|Texas Instruments Incorporated
|16-Channel LED Driver w/EEprom DOT Correction & Grayscale PWM Control
| Marketing part#   Digital Voltage Range   Package-type   #pins
| TLC5940NT   3.0 to 5.5V   PDIP   28
| TLC5940NTG4   3.0 to 5.5V   PDIP   28
| TLC5940PWP   3.0 to 5.5V   HTSSOP   28
| TLC5940PWPG4   3.0 to 5.5V   HTSSOP   28
| TLC5940PWPR   3.0 to 5.5V   HTSSOP   28
| TLC5940PWPRG4   3.0 to 5.5V   HTSSOP   28
| TLC5940RHBR   3.0 to 5.5V   QFN   32
| TLC5940RHBRG4   3.0 to 5.5V   QFN   32
[IBIS Ver]   3.2
[File name]   tlc5940.ibs
|SIMDE Ver   V2.0 - 201002 - RHL4 - Build 372
[File Rev]   1.0
[Date]   9/8/2010
[Source]
| Texas Instruments Incorporated.
| Analog-eLab Design Center, HPA
| 12500 TI Blvd
| Dallas, TX -75243
| e-mail: elab_ibis@list.ti.com
| -Model generated from simulations in TISPICE
[Notes]   Revision History:
| Rev 1.0: 9/8/2010
| - Initial version of the model
| - Model generated from simulations in TISPICE
| - Model matched to SPICE simulation
| - C_comp although listed in numerical order of value are
|   obtained from varying PVT conditions. For PVT conditions for
|   each specific value refer the buffer description under
|   respective [Model]. IBIS model user is responsible for using
|   appropriate C_comp to simulate for Signal Integrity.
[Disclaimer]
| This model is designed as an aid for customers of Texas Instruments.
| TI and its licensors and suppliers make no warranties, either expressed
| or implied, with respect to this  model, including the warranties of
| merchantability or fitness for a particular purpose. The model is
| provided solely on an "as is" basis. The entire risk as to its quality
| and performance is with the customer.
[Copyright]
 (C) Copyright 2010 Texas Instruments Incorporated.All rights reserved.
|   TLC5940PWP
[Component]   TLC5940PWP
[Manufacturer]   TI
[Package]   |28 HTSSOP -  PWP package
|   typ   min   max
R_pkg   0.08193   0.05437   0.11416
L_pkg   2.86912nH   2.09991nH   4.18774nH
C_pkg   0.49015pF   0.4277pF   0.62179pF
[Pin]  signal_name   model_name   R_pin   L_pin   C_pin
1   GND   GND   0.04408   3.68717nH  0.70954pF
2   BLANK   INPUT   0.11352   3.84749nH  0.5889pF
3   XLAT   INPUT   0.09801   3.15255nH  0.48789pF
4   SCLK   INPUT   0.08218   2.76394nH  0.47901pF
5   SIN   INPUT   0.06987   2.46426nH  0.45688pF
6   VPRG   TERM   0.06162   2.27164nH  0.43906pF
7   OUT0   TERM   0.05581   2.13231nH  0.42984pF
8   OUT1   TERM   0.05437   2.09991nH  0.42781pF
9   OUT2   TERM   0.05967   2.23421nH  0.43955pF
10   OUT3   TERM   0.06917   2.45494nH  0.45622pF
11   OUT4   TERM   0.08271   2.78637nH  0.47877pF
12   OUT5   TERM   0.09792   3.16124nH  0.48694pF
13   OUT6   TERM   0.11416   3.87798nH  0.58872pF
14   OUT7   TERM   0.11147   4.18774nH  0.62179pF
15   OUT8   TERM   0.11145   4.18614nH  0.62137pF
16   OUT9   TERM   0.11411   3.87312nH  0.58858pF
17   OUT10   TERM   0.09792   3.16127nH  0.48694pF
18   OUT11   TERM   0.08271   2.78627nH  0.4788pF
19   OUT12   TERM   0.06917   2.45496nH  0.45621pF
20   OUT13   TERM   0.05967   2.23422nH  0.43953pF
21   OUT14   TERM   0.05437   2.10017nH  0.4277pF
22   OUT15   TERM   0.05581   2.13233nH  0.42914pF
23   XERR   XERR   0.06071   2.24986nH  0.43618pF
24   SOUT   OUTPUT   0.06752   2.4073nH   0.45212pF
25   GSCLK   INPUT   0.07954   2.69933nH  0.47442pF
26   DCPRG   INPUT   0.09534   3.08672nH  0.48741pF
27   IREF   TERM   0.11132   3.79072nH  0.58402pF
28   VCC   POWER   0.1141   4.23499nH  0.6181pF
|   TLC5940RHB
[Component]   TLC5940RHB
[Manufacturer]   TI
[Package]   |32 QFN -  RHB package
|   typ   min   max
R_pkg   0.08145   0.00024   0.10927
L_pkg   1.45259nH   0.05657nH   1.97475nH
C_pkg   0.13023pF   0.04173pF   0.1566pF
[Pin]  signal_name   model_name   R_pin   L_pin   C_pin
1   SCLK   INPUT   0.10683   1.92034nH  0.15309pF
2   SIN   INPUT   0.10002   1.78371nH  0.15428pF
3   VPRG   TERM   0.09526   1.68977nH  0.14836pF
4   OUT0   TERM   0.09177   1.62167nH  0.14501pF
5   OUT1   TERM   0.09085   1.60457nH  0.14424pF
6   OUT2   TERM   0.0945   1.67768nH  0.14872pF
7   OUT3   TERM   0.10082   1.8039nH   0.1566pF
8   OUT4   TERM   0.10927   1.97475nH  0.15632pF
9   OUT5   TERM   0.10077   1.80744nH  0.14432pF
10   OUT6   TERM   0.0827   1.44881nH  0.13242pF
11   OUT7   TERM   0.07284   1.25667nH  0.11872pF
12   NC   NC   0.00024   0.05657nH  0.04173pF
13   NC   NC   0.00024   0.05657nH  0.04173pF
14   OUT8   TERM   0.07284   1.25667nH  0.11872pF
15   OUT9   TERM   0.0827   1.4489nH   0.13243pF
16   OUT10   TERM   0.10077   1.80745nH  0.14432pF
17   OUT11   TERM   0.10927   1.97474nH  0.15632pF
18   OUT12   TERM   0.10082   1.80391nH  0.1566pF
19   OUT13   TERM   0.0945   1.67767nH  0.14871pF
20   OUT14   TERM   0.09085   1.60457nH  0.14418pF
21   OUT15   TERM   0.09177   1.62167nH  0.14416pF
22   XERR   XERR   0.09456   1.67617nH  0.14589pF
23   SOUT   OUTPUT   0.09812   1.7463nH   0.15114pF
24   GSCLK   INPUT   0.10453   1.87495nH  0.15048pF
25   DCPRG   INPUT   0.09727   1.72964nH  0.14393pF
26   IREF   TERM   0.07733   1.33561nH  0.12703pF
27   VCC   POWER   0.07581   1.30567nH  0.11952pF
28   NC   NC   0.00024   0.05657nH  0.04173pF
29   NC   NC   0.00024   0.05657nH  0.04173pF
30   GND   GND   0.026   0.97478nH  0.17132pF
31   BLANK   INPUT   0.08126   1.4124nH   0.13077pF
32   XLAT   INPUT   0.10039   1.79135nH  0.1433pF
|   TLC5940NT
[Component]   TLC5940NT
[Manufacturer]   TI
[Package]   |28 PDIP - NT package
|   typ   min   max
R_pkg   0.09933   0.05587   0.11678
L_pkg   9.80714nH   4.19963nH   14.18524nH
C_pkg   1.93393pF   0.79043pF   2.82131pF
[Pin]  signal_name   model_name   R_pin   L_pin   C_pin
1   OUT1   TERM   0.1159   14.13964nH 2.62594pF
2   OUT2   TERM   0.11473   12.46205nH 2.82091pF
3   OUT3   TERM   0.11478   11.24633nH 2.48874pF
4   OUT4   TERM   0.11446   9.34358nH  1.7845pF
5   OUT5   TERM   0.09096   8.21191nH  1.39011pF
6   OUT6   TERM   0.07072   6.33623nH  1.07636pF
7   OUT7   TERM   0.05587   4.19963nH  0.79043pF
8   OUT8   TERM   0.05587   4.20123nH  0.79048pF
9   OUT9   TERM   0.07073   6.34383nH  1.07657pF
10   OUT10   TERM   0.09096   8.222nH   1.39055pF
11   OUT11   TERM   0.11446   9.35772nH  1.78486pF
12   OUT12   TERM   0.11478   11.26061nH 2.48922pF
13   OUT13   TERM   0.11473   12.47694nH 2.82131pF
14   OUT14   TERM   0.1159   14.15458nH 2.6263pF
15   OUT15   TERM   0.11678   14.18524nH 2.62492pF
16   XERR   XERR   0.11459   12.47163nH 2.81415pF
17   SOUT   OUTPUT   0.11285   11.19313nH 2.48003pF
18   GSCLK   INPUT   0.11118   9.24258nH  1.77765pF
19   DCPRG   INPUT   0.08832   8.13519nH  1.38911pF
20   IREF   TERM   0.06641   6.19973nH  1.07016pF
21   VCC   POWER   0.05808   4.27313nH  0.79299pF
22   GND   GND   0.02264   3.87899nH  0.85343pF
23   BLANK   INPUT   0.06962   6.29993nH  1.07492pF
24   XLAT   INPUT   0.09008   8.18201nH  1.38803pF
25   SCLK   INPUT   0.11228   9.26739nH  1.77903pF
26   SIN   INPUT   0.11379   11.21171nH 2.48315pF
27   VPRG   TERM   0.11496   12.47044nH 2.81809pF
28   OUT0   TERM   0.11678   14.17048nH 2.6267pF
|   Model Selectors
[Model Selector] INPUT
input_3p3v   3.3V digital input
input_5p0v   5.0V digital input
[Model Selector] OUTPUT
output_3p3v   3.3V digital output
output_5p0v   5.0V digital output
[Model Selector] XERR
xerr_3p3v   3.3V output_open_drain
xerr_5p0v   5.0V output_open_drain
[Model Selector] TERM
term_3-3V  3.3V nominal termination
term_5-0V  5.0V nominal termination
[Model] term_3-3V
Model_type Terminator
C_comp   1.0e-20F  1.0e-20F  1.0e-20F
|   typ   min   max
[Voltage Range]   3.3V   3.0V   3.6V
[POWER Clamp Reference]   3.3V   3.0V   3.6V
[GND Clamp Reference]   0V   0V   0V
|Ambient Temperature   25   85   -40
|Junction Temperature
[Temperature Range]   65   125   -40
[Model] term_5-0V
Model_type Terminator
C_comp   1.0e-20F  1.0e-20F  1.0e-20F
|   typ   min   max
[Voltage Range]   5.0V   4.5V   5.5V
[POWER Clamp Reference]   5.0V   4.5V   5.5V
[GND Clamp Reference]   0V   0V   0V
|Ambient Temperature   25   85   -40
|Junction Temperature
[Temperature Range]   65   125   -40
| Models and submodels in the file (8): input_3p3v (Input), input_5p0v (Input), output_3p3v (Output), output_5p0v (Output), xerr_3p3v (Open_drain), xerr_5p0v (Open_drain), term_3-3V (Terminator), term_5-0V (Terminator)
